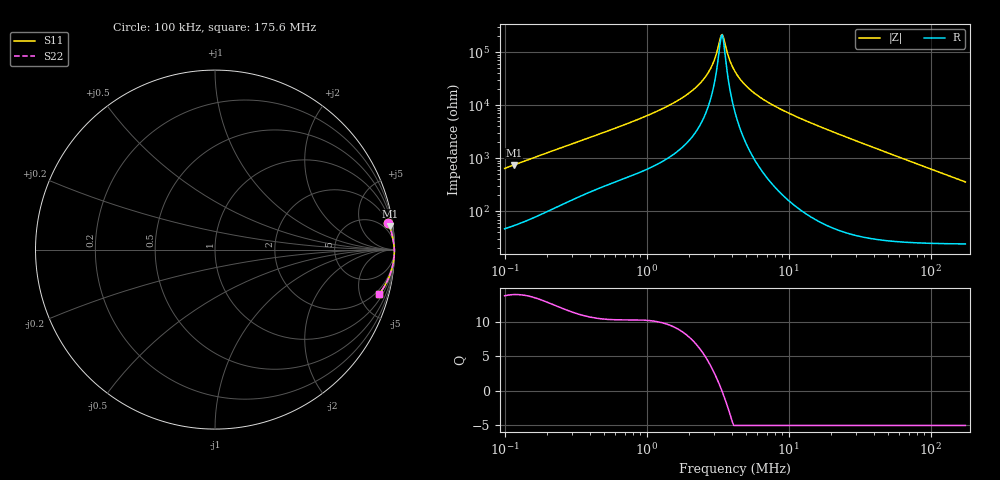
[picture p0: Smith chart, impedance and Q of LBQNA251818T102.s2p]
! LBQNA251818T102  S-PARAMETER MODEL  ( General Type )
! Model Generated by TAIYO YUDEN Corporation (http://www.ty-top.com)
! Version 1.0
! TAIYO YUDEN Control No. 191025NI43SB-FBB
! Copyright(c) 2019 TAIYO YUDEN CO.,LTD. All Rights Reserved.
! Product Description (link to TY-COMPAS)
! https://ds.yuden.co.jp/TYCOMPAS/or/detail?pn=LBQNA251818T102K&u=M
! Products Name : Inductors
! Characteristics :
!  Inductance : 1000 uH , SRF(min) : 2.4 MHz , DC Resistance(max) : 31.2 Ohm
!  Rated Current : Saturation :25 mA , Temp Rise : 45 mA (20 degC)
!  Case Size : 2.5 x 1.8 / 0.098 x 0.071 [mm/inch] , Thickness : 1.8 / 0.071 [mm/inch]
!  (Conditions: Temperature = 25 degC , DC Bias Current/Voltage = 0A / 0V)
! External Node Assignments :
!  1  o---GGG---o  2
! GND o---------o GND
! Frequency Range : 0.1MHz  -  175.64884MHz  [ 402 STEP ]
# MHz S RI R 50
! Freq[MHz].  S11 Real  S11 Imag  S21 Real  S21 Imag  S12 Real  S12 Imag  S22 Real  S22 Imag
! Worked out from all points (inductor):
!   401 points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, 100 kHz to 175.6 MHz, reference 50 ohm
!   read as one part in series: L = 1.02 mH near 103.8 kHz
!   highest Q = 13.9 at 116.1 kHz (marker M1), where L = 1.02 mH
!   self-resonance near 3.35 MHz
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0.1  0.9662 0.1479  0.0338 -0.1479  0.0338 -0.1479  0.9662 0.1479
0.116116  0.9734 0.1288  0.0266 -0.1288  0.0266 -0.1288  0.9734 0.1288
0.349525  0.9938 0.0453  0.00624 -0.0453  0.00624 -0.0453  0.9938 0.0453
0.751717  0.9974 0.0214  0.00256 -0.0214  0.00256 -0.0214  0.9974 0.0214
1.221676  0.9986 0.0124  0.00141 -0.0124  0.00141 -0.0124  0.9986 0.0124
1.842518  0.9991 0.00679  0.000862 -0.00679  0.000862 -0.00679  0.9991 0.00679
2.438293  0.9994 0.00355  0.000632 -0.00355  0.000632 -0.00355  0.9994 0.00355
2.676973  0.9994 0.00253  0.000574 -0.00253  0.000574 -0.00253  0.9994 0.00253
2.884632  0.9995 0.00172  0.000533 -0.00172  0.000533 -0.00172  0.9995 0.00172
3.050881  0.9995 0.00112  0.000506 -0.00112  0.000506 -0.00112  0.9995 0.00112
3.287545  0.9995 0.000327  0.000474 -0.000327  0.000474 -0.000327  0.9995 0.000327
3.349525  0.9995 0.000128  0.000467 -0.000128  0.000467 -0.000128  0.9995 0.000128
3.477015  0.9995 -0.000271  0.000453 0.000271  0.000453 0.000271  0.9995 -0.000271
3.889343  0.9996 -0.00147  0.000418 0.00147  0.000418 0.00147  0.9996 -0.00147
4.270063  0.9996 -0.00249  0.000397 0.00249  0.000397 0.00249  0.9996 -0.00249
5.051714  0.9996 -0.0044  0.000374 0.0044  0.000374 0.0044  0.9996 -0.0044
6.440058  0.9996 -0.00739  0.000377 0.00739  0.000377 0.00739  0.9996 -0.00739
9.01361  0.9995 -0.0123  0.000464 0.0123  0.000464 0.0123  0.9995 -0.0123
14.64875  0.9991 -0.0221  0.000858 0.0221  0.000858 0.0221  0.9991 -0.0221
51.20104  0.9916 -0.0805  0.00836 0.0805  0.00836 0.0805  0.9916 -0.0805
104.1166  0.967 -0.1591  0.033 0.1591  0.033 0.1591  0.967 -0.1591
175.6488  0.913 -0.2499  0.087 0.2499  0.087 0.2499  0.913 -0.2499
